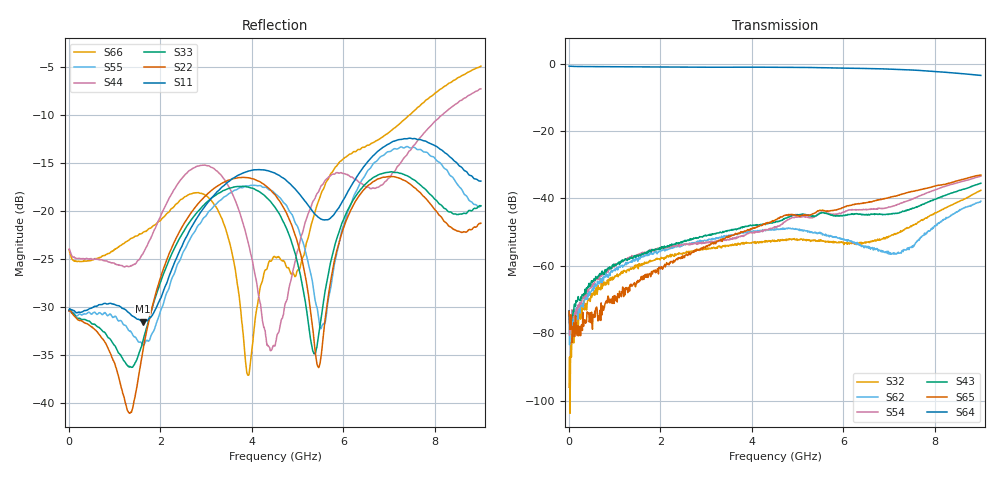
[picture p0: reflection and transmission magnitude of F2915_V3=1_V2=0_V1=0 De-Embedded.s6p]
! Integrated Device Technology
! Corporate Headquarters
! 6024 Silver Creek Valley Road
! San Jose, CA 95138  USA
! Phone:  1-408-284-8200
! Toll Free:  1-800-223-1366
! Webpage:  http://www.idt.com/
! Timing and RF Division
! 515 Groton Road, Suite 102
! Westford, MA 01886-6024
! Device:  F2915
! Description: High Reliability SP5T RF Switch
! Frequency:  0.05 -  8.GHz
! Package:  4x4 mm Thin QFN Plastic Package: 24 pin
! Ports:  6 RF,  5 DC
!  Pin  1  = GND
!  Pin  2  = RF5  =  Port 5
!  Pin  3  = GND
!  Pin  4  = GND
!  Pin  5  = RF4  =  Port 4
!  Pin  6  = GND
!  Pin  7  = GND
!  Pin  8  = RF3  =  Port 3
!  Pin  9  = GND
!  Pin 10  = GND
!  Pin 11  = RF2  =  Port 2
!  Pin 12  = GND
!  Pin 13  = GND
!  Pin 14  = RF1  =  Port 1
!  Pin 15  = GND
!  Pin 16  = Vcc
!  Pin 17  = V1
!  Pin 18  = V2
!  Pin 19  = V3
!  Pin 20  = VSSext
!  Pin 21  = GND
!  Pin 22  = RFC  =  Port 6
!  Pin 23  = GND
!  Pin 24  = GND
! Voltage:  VDD  =  +3.30 Volts
!  VSSEXT =  0.00 Volts
! Current:  IDD  = 253  uA
! State:  RF4 Selected
! V1:  Logic LOW
! V2:  Logic LOW
! V3:  Logic HIGH
! Data:  The device was measured on the F291x evaluation board which has
!  individual transmission lines to the RF pins.  Data was collected
!  using a calibrated network analyzer.  The input lines were
!  modeled using Automatic Fixture Removal (AFR) from Keysight.
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# Hz S  dB  R 50
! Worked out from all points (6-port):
!   900 points, 10 MHz to 9 GHz, reference 50 ohm
!   strongest paths, dB at 10 MHz, 2.26 GHz, 4.51 GHz, 6.76 GHz, 9 GHz:
!     S64: -0.8, -1.1, -1.1, -1.5, -3.5
!     S65: -73.5, -58.8, -46.4, -40.5, -33.1
!     S43: -73.3, -53.8, -47.0, -44.8, -35.5
!     S54: -74.1, -54.2, -48.4, -42.9, -33.4
!     S62: -74.0, -54.8, -49.1, -55.6, -40.8
!     S32: -96.0, -56.6, -52.7, -52.4, -37.6
!   lowest |S11| = -31.5 dB at 1.62 GHz (marker M1), VSWR 1.05, Z = 49.5 + j2.61 ohm
!   |S11| at or under -10 dB: start of sweep to end of sweep
